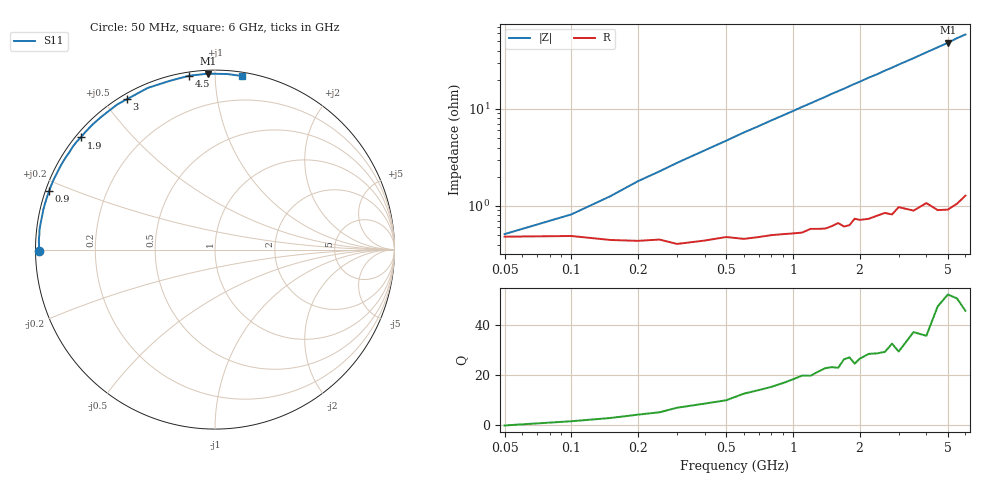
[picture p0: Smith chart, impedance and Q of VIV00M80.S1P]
! Infineon Technologies  Discrete & RF Semiconductors
! BB 804
! Si Tuning Diode in SOT23
! VR =
! S-Parameters:  July  1999
# GHz  S  MA  R  50
!  f  S11
! GHz  MAG  ANG
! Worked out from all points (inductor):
!   34 points, 50 MHz to 6 GHz, reference 50 ohm
!   read as one part to ground: L = 1.42 nH near 200 MHz
!   highest Q = 50.9 at 5 GHz (marker M1), where L = 1.53 nH
!   S11 on the Smith chart (normalised r, x): 50 MHz: 0.01, -0.00; 900 MHz: 0.01, +0.17; 1.9 GHz: 0.01, +0.36; 3 GHz: 0.02, +0.57; 4.5 GHz: 0.02, +0.86; 6 GHz: 0.03, +1.17
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0.05  0.9809 -179.6
0.1  0.9806 178.5
0.2  0.9827 176.0
0.3  0.9839 173.7
0.4  0.9827 171.5
0.6  0.9821 167.0
0.8  0.9806 162.7
0.9  0.9803 160.6
1.1  0.9798 156.3
1.3  0.9784 152.2
1.4  0.9784 150.2
1.5  0.9774 148.0
1.6  0.9759 146.1
1.7  0.978 144.2
1.8  0.9776 142.1
1.9  0.9742 140.1
2  0.9752 138.3
2.2  0.9752 134.4
2.4  0.974 131.0
2.6  0.9732 127.2
2.8  0.9749 123.9
3  0.9711 120.4
3.5  0.9755 112.6
4  0.9734 105.1
4.5  0.9795 98.4
5  0.9811 92.3
5.5  0.9806 86.0
6  0.9787 81.0
